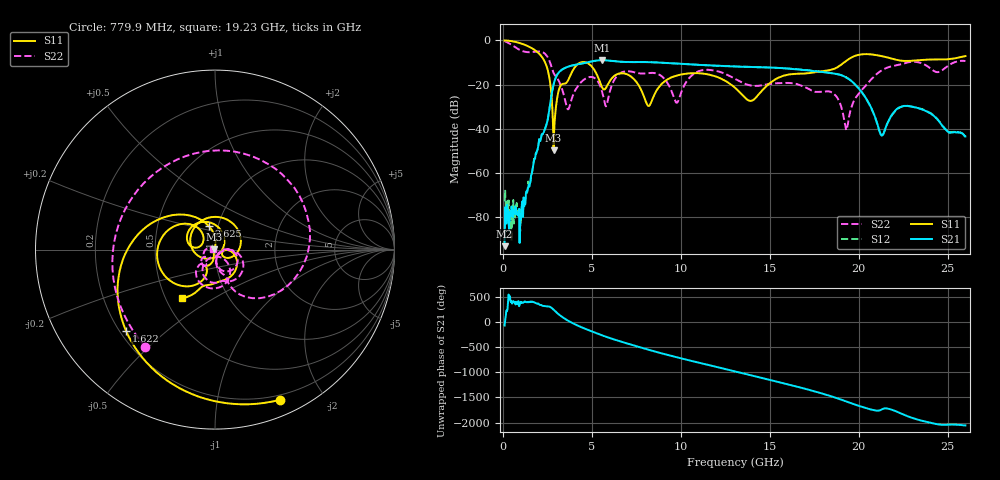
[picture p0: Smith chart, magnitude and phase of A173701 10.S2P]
!  2-Port S-parameters saved by WinCal
! VAR MeasName=S-Parameters (CALIBRATED_DATA) read from VNA (N5245A)
! VAR MeasDate=2017-6-7 10:29:04
! VAR NAME=A173701 10
! VAR FILENAME=A173701 10.S2P
! VAR DATE=2017-6-7 10:29:04
! VAR PHYS_PORTS=1,2
# Hz S DB R 50
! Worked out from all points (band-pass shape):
!   801 points, 100 MHz to 26 GHz, reference 50 ohm
!   highest |S21| = -8.89 dB at 5.571 GHz (marker M1); lowest = -93.0 dB at 100 MHz (marker M2)
!   |S21| within 3 dB of the highest: 3.656 GHz to 13.3 GHz (9.646 GHz wide, 114 % of centre); 13.38593 GHz to 13.44267 GHz (56.74 MHz wide, 0.423 % of centre)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
!   lowest |S11| = -49.7 dB at 2.852 GHz (marker M3), VSWR 1.01, Z = 49.7 + j0.171 ohm
!   |S11| at or under -10 dB: 2.378 GHz to 4.361 GHz (1.983 GHz wide, 58.9 % of centre); 4.693 GHz to 19.18 GHz (14.48 GHz wide, 121 % of centre)
!   |S22| runs from -40.5 to -0.3 dB; largest |S21 - S12| = 0.0042
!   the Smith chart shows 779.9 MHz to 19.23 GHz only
!   S11 on the Smith chart (normalised r, x): 779.9 MHz: 0.15, -1.51; 1.622 GHz: 0.23, -0.37; 2.625 GHz: 0.90, +0.24; 19.23 GHz: 0.60, -0.37
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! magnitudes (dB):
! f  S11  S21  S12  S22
! 100 MHz  0.0  -93.0  -72.6  -0.3
! 779.9 MHz  -0.8  -78.5  -73.4  -3.5
! 1.622 GHz  -3.5  -60.5  -60.2  -5.3
! 2.625 GHz  -17.3  -30.7  -30.8  -9.3
! 2.852 GHz  -49.7  -19.9  -19.9  -14.7
! 3.661 GHz  -18.1  -11.9  -11.9  -31.1
! 4.438 GHz  -9.8  -10.4  -10.4  -18.5
! 5.571 GHz  -21.0  -8.9  -8.9  -22.9
! 6.963 GHz  -15.3  -9.7  -9.8  -13.9
! 8.194 GHz  -29.6  -9.8  -9.8  -14.7
! 8.744 GHz  -21.4  -10.0  -10.0  -15.3
! 9.78 GHz  -15.8  -10.4  -10.5  -28.2
! 11.01 GHz  -14.8  -11.0  -11.1  -13.9
! 13.05 GHz  -21.4  -11.8  -11.8  -17.4
! 13.96 GHz  -27.3  -12.0  -12.0  -20.4
! 17.39 GHz  -14.6  -13.8  -13.7  -22.7
! 18.65 GHz  -12.8  -15.0  -15.0  -24.5
! 19.23 GHz  -9.6  -16.5  -16.3  -37.9
! 21.27 GHz  -7.0  -42.9  -42.9  -13.7
! 21.69 GHz  -7.9  -36.1  -36.3  -12.0
! 23.05 GHz  -9.1  -30.0  -30.0  -9.7
! 26 GHz  -7.1  -43.4  -43.6  -9.3
